(* Logix 5000 AddOnInstructionDefinition export Banner_Analog_Converter_PD_v4; software revision 33.00 *)

TYPE Banner_Analog_Converter_PDIO_v4 :
STRUCT
   S15C_UI : Banner_S15C_UI_PDI_v4;
   R45C_UI : Banner_R45C_UI_PD_v4;
   R45C_UUII : Banner_R45C_UU_II_PD_v4;
   DTI : SINT[8];
   DTO : SINT[8];
END_STRUCT
END_TYPE

TYPE Banner_R45C_Set_0_v4 :
STRUCT
   Measurement : DINT;
   Analog_Output : DINT;
END_STRUCT
END_TYPE

TYPE Banner_R45C_Set_1_v4 :
STRUCT
   Measurement : DINT;
   Scale : INT;
   Analog_Output : DINT;
END_STRUCT
END_TYPE

TYPE Banner_R45C_UI_PD_v4 :   // UDT with all of the variables needed to control an IO-Link R45C U or R45C I.
STRUCT
   Data_Set_0 : Banner_R45C_Set_0_v4;
   Data_Set_1 : Banner_R45C_Set_1_v4;
END_STRUCT
END_TYPE

TYPE Banner_R45C_UU_II_PD_v4 :   // UDT with all of the variables needed to control an IO-Link R45C UU or R45C II.
STRUCT
   Data_0 : Banner_R45C_UUII_Set_0_v4;
   Data_1 : Banner_R45C_UUII_Set_1_v4;
END_STRUCT
END_TYPE

TYPE Banner_R45C_UUII_Set_0_v4 :
STRUCT
   Measurement_1 : DINT;
   Measurement_2 : DINT;
   Analog_Output_1 : DINT;
   Analog_Output_2 : DINT;
END_STRUCT
END_TYPE

TYPE Banner_R45C_UUII_Set_1_v4 :
STRUCT
   Measurement_1 : DINT;
   Scale_1 : INT;
   SSC1_Switching_Signal : DINT;
   Measurement_2 : DINT;
   Scale_2 : INT;
   SSC2_Switching_Signal : DINT;
   Analog_Output_1 : DINT;
   Analog_Output_2 : DINT;
END_STRUCT
END_TYPE

TYPE Banner_S15C_UI_PDI_v4 :   // UDT with all of the variables needed to control an IO-Link S15C U or S15C I.
STRUCT
   Data_Set_0 : Banner_S15C_UI_Set_0_v4;
   Data_Set_1 : Banner_S15C_UI_Set_1_v4;
END_STRUCT
END_TYPE

TYPE Banner_S15C_UI_Set_0_v4 :
STRUCT
   Measurement : DINT;
END_STRUCT
END_TYPE

TYPE Banner_S15C_UI_Set_1_v4 :
STRUCT
   Measurement : DINT;   // Current or Voltage values
   Scale : INT;   // 250 = microAmps, 253 = microVolts
END_STRUCT
END_TYPE

ADD_ON_INSTRUCTION Banner_Analog_Converter_PD_v4   (* revision 4.0, vendor Banner Engineering *)
// AOI that used with the S15C UI, R45C U/I, and R45C UU/II sensor.
VAR_IN_OUT
   PD : Banner_Analog_Converter_PDIO_v4; {required}
END_VAR
VAR_INPUT
   Byte_Swap : BOOL; {required}
   Data_Set : SINT; {required}
   Type : SINT; {required}
END_VAR
VAR
   TempOut : SINT[8]; {access None}
   TempIn : SINT[8]; {access None}
END_VAR

ROUTINE Logic   (* ladder *)
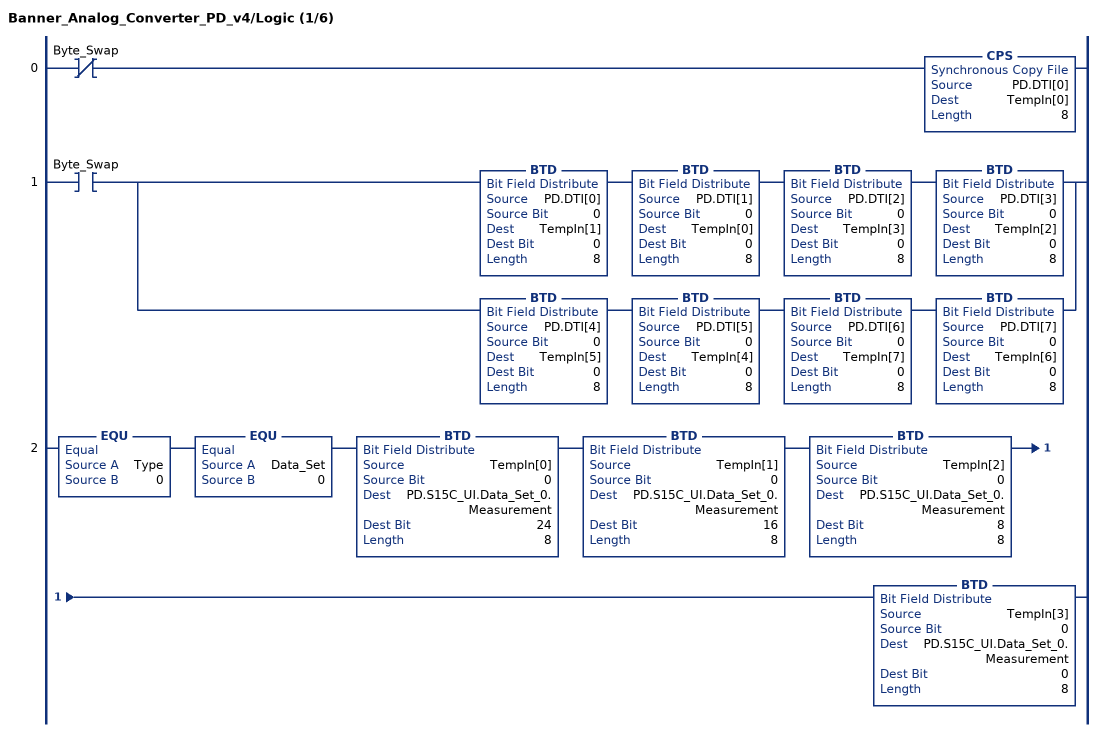
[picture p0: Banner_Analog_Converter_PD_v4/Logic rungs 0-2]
   0: XIO(Byte_Swap)CPS(PD.DTI[0],TempIn[0],8);
   1: XIC(Byte_Swap)[BTD(PD.DTI[0],0,TempIn[1],0,8) BTD(PD.DTI[1],0,TempIn[0],0,8) BTD(PD.DTI[2],0,TempIn[3],0,8) BTD(PD.DTI[3],0,TempIn[2],0,8) ,BTD(PD.DTI[4],0,TempIn[5],0,8) BTD(PD.DTI[5],0,TempIn[4],0,8) BTD(PD.DTI[6],0,TempIn[7],0,8) BTD(PD.DTI[7],0,TempIn[6],0,8) ];
   2: EQU(Type,0)EQU(Data_Set,0)BTD(TempIn[0],0,PD.S15C_UI.Data_Set_0.Measurement,24,8)BTD(TempIn[1],0,PD.S15C_UI.Data_Set_0.Measurement,16,8)BTD(TempIn[2],0,PD.S15C_UI.Data_Set_0.Measurement,8,8)BTD(TempIn[3],0,PD.S15C_UI.Data_Set_0.Measurement,0,8);
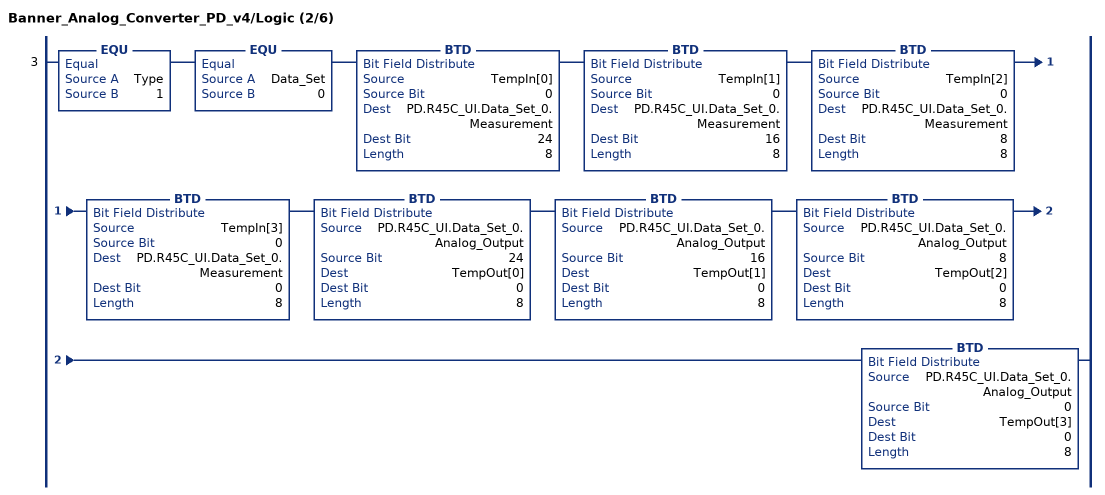
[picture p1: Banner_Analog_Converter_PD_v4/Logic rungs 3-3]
   3: EQU(Type,1)EQU(Data_Set,0)BTD(TempIn[0],0,PD.R45C_UI.Data_Set_0.Measurement,24,8)BTD(TempIn[1],0,PD.R45C_UI.Data_Set_0.Measurement,16,8)BTD(TempIn[2],0,PD.R45C_UI.Data_Set_0.Measurement,8,8)BTD(TempIn[3],0,PD.R45C_UI.Data_Set_0.Measurement,0,8)BTD(PD.R45C_UI.Data_Set_0.Analog_Output,24,TempOut[0],0,8)BTD(PD.R45C_UI.Data_Set_0.Analog_Output,16,TempOut[1],0,8)BTD(PD.R45C_UI.Data_Set_0.Analog_Output,8,TempOut[2],0,8)BTD(PD.R45C_UI.Data_Set_0.Analog_Output,0,TempOut[3],0,8);
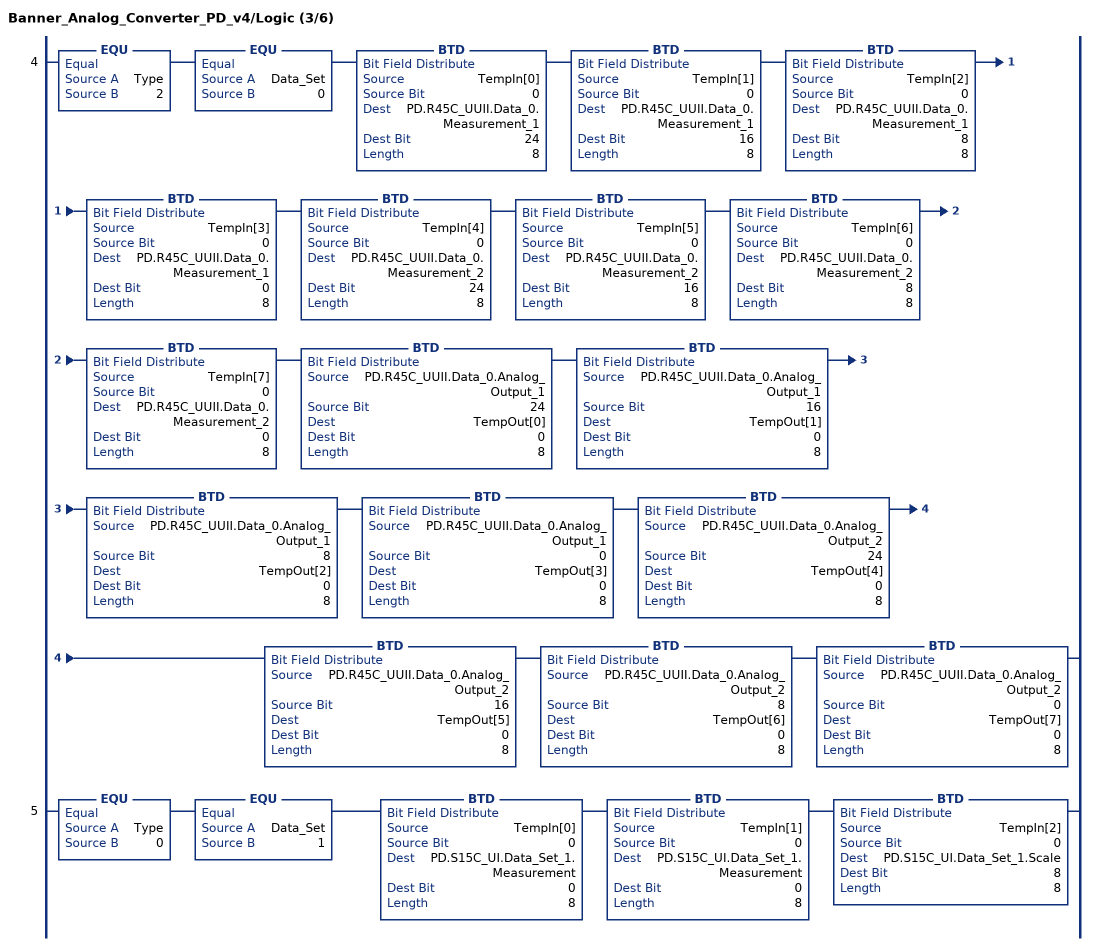
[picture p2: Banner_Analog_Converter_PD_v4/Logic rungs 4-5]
   4: EQU(Type,2)EQU(Data_Set,0)BTD(TempIn[0],0,PD.R45C_UUII.Data_0.Measurement_1,24,8)BTD(TempIn[1],0,PD.R45C_UUII.Data_0.Measurement_1,16,8)BTD(TempIn[2],0,PD.R45C_UUII.Data_0.Measurement_1,8,8)BTD(TempIn[3],0,PD.R45C_UUII.Data_0.Measurement_1,0,8)BTD(TempIn[4],0,PD.R45C_UUII.Data_0.Measurement_2,24,8)BTD(TempIn[5],0,PD.R45C_UUII.Data_0.Measurement_2,16,8)BTD(TempIn[6],0,PD.R45C_UUII.Data_0.Measurement_2,8,8)BTD(TempIn[7],0,PD.R45C_UUII.Data_0.Measurement_2,0,8)BTD(PD.R45C_UUII.Data_0.Analog_Output_1,24,TempOut[0],0,8)BTD(PD.R45C_UUII.Data_0.Analog_Output_1,16,TempOut[1],0,8)BTD(PD.R45C_UUII.Data_0.Analog_Output_1,8,TempOut[2],0,8)BTD(PD.R45C_UUII.Data_0.Analog_Output_1,0,TempOut[3],0,8)BTD(PD.R45C_UUII.Data_0.Analog_Output_2,24,TempOut[4],0,8)BTD(PD.R45C_UUII.Data_0.Analog_Output_2,16,TempOut[5],0,8)BTD(PD.R45C_UUII.Data_0.Analog_Output_2,8,TempOut[6],0,8)BTD(PD.R45C_UUII.Data_0.Analog_Output_2,0,TempOut[7],0,8);
   5: EQU(Type,0)EQU(Data_Set,1)BTD(TempIn[0],0,PD.S15C_UI.Data_Set_1.Measurement,0,8)BTD(TempIn[1],0,PD.S15C_UI.Data_Set_1.Measurement,0,8)BTD(TempIn[2],0,PD.S15C_UI.Data_Set_1.Scale,8,8);
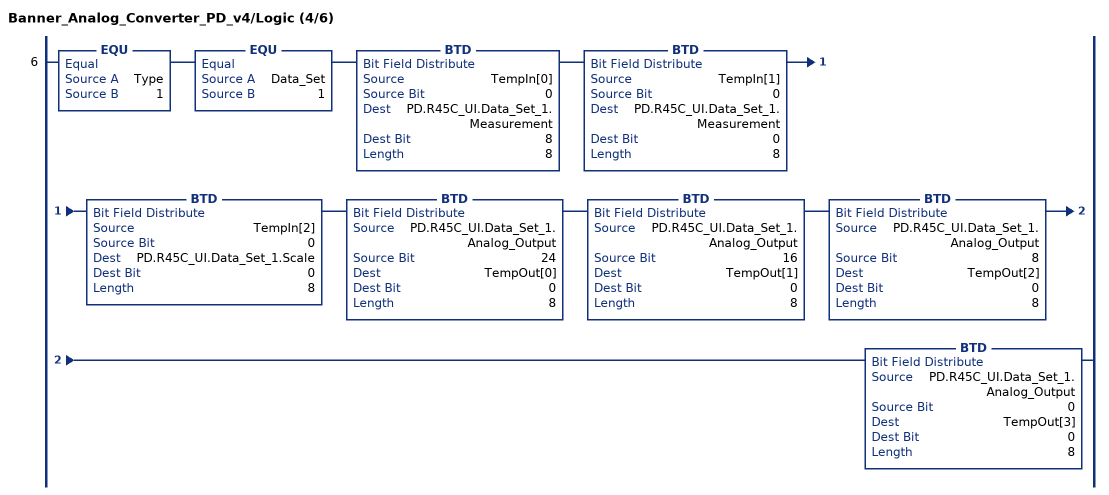
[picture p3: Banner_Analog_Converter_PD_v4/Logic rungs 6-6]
   6: EQU(Type,1)EQU(Data_Set,1)BTD(TempIn[0],0,PD.R45C_UI.Data_Set_1.Measurement,8,8)BTD(TempIn[1],0,PD.R45C_UI.Data_Set_1.Measurement,0,8)BTD(TempIn[2],0,PD.R45C_UI.Data_Set_1.Scale,0,8)BTD(PD.R45C_UI.Data_Set_1.Analog_Output,24,TempOut[0],0,8)BTD(PD.R45C_UI.Data_Set_1.Analog_Output,16,TempOut[1],0,8)BTD(PD.R45C_UI.Data_Set_1.Analog_Output,8,TempOut[2],0,8)BTD(PD.R45C_UI.Data_Set_1.Analog_Output,0,TempOut[3],0,8);
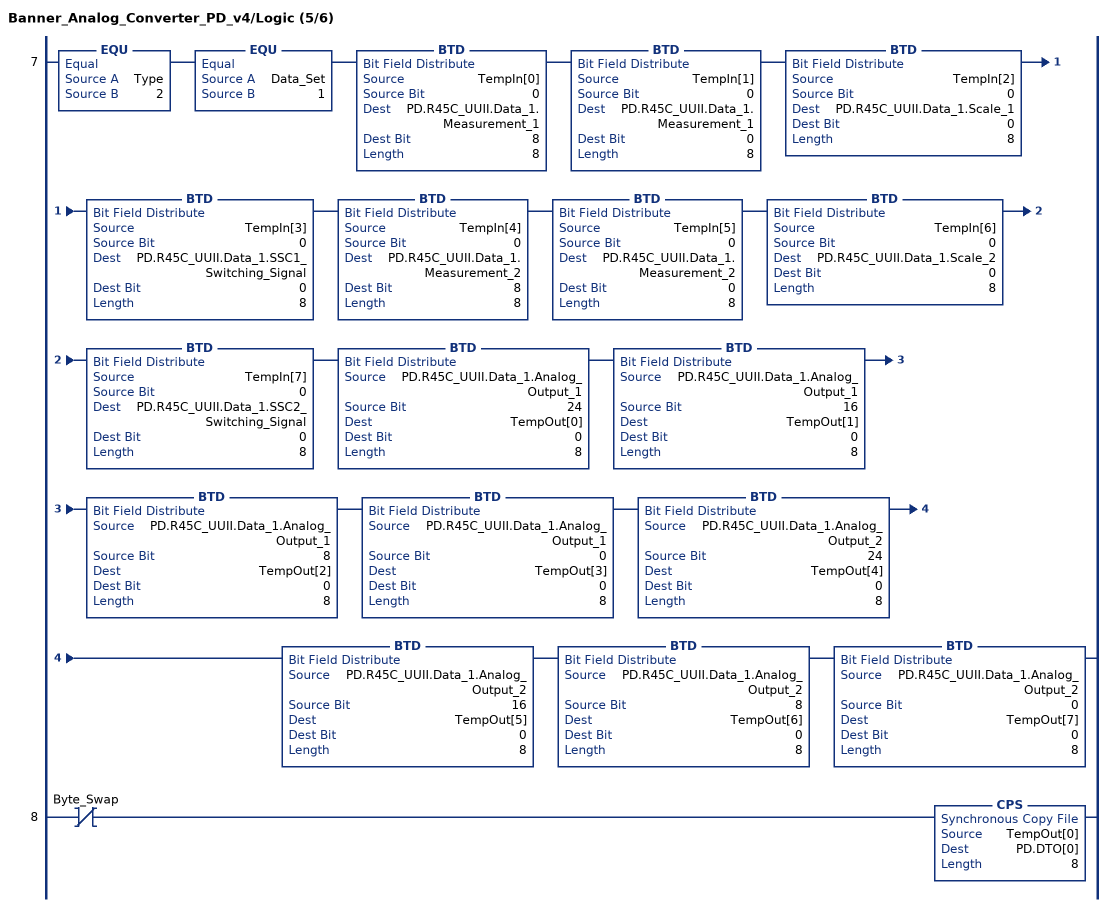
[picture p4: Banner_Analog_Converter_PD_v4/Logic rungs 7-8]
   7: EQU(Type,2)EQU(Data_Set,1)BTD(TempIn[0],0,PD.R45C_UUII.Data_1.Measurement_1,8,8)BTD(TempIn[1],0,PD.R45C_UUII.Data_1.Measurement_1,0,8)BTD(TempIn[2],0,PD.R45C_UUII.Data_1.Scale_1,0,8)BTD(TempIn[3],0,PD.R45C_UUII.Data_1.SSC1_Switching_Signal,0,8)BTD(TempIn[4],0,PD.R45C_UUII.Data_1.Measurement_2,8,8)BTD(TempIn[5],0,PD.R45C_UUII.Data_1.Measurement_2,0,8)BTD(TempIn[6],0,PD.R45C_UUII.Data_1.Scale_2,0,8)BTD(TempIn[7],0,PD.R45C_UUII.Data_1.SSC2_Switching_Signal,0,8)BTD(PD.R45C_UUII.Data_1.Analog_Output_1,24,TempOut[0],0,8)BTD(PD.R45C_UUII.Data_1.Analog_Output_1,16,TempOut[1],0,8)BTD(PD.R45C_UUII.Data_1.Analog_Output_1,8,TempOut[2],0,8)BTD(PD.R45C_UUII.Data_1.Analog_Output_1,0,TempOut[3],0,8)BTD(PD.R45C_UUII.Data_1.Analog_Output_2,24,TempOut[4],0,8)BTD(PD.R45C_UUII.Data_1.Analog_Output_2,16,TempOut[5],0,8)BTD(PD.R45C_UUII.Data_1.Analog_Output_2,8,TempOut[6],0,8)BTD(PD.R45C_UUII.Data_1.Analog_Output_2,0,TempOut[7],0,8);
   8: XIO(Byte_Swap)CPS(TempOut[0],PD.DTO[0],8);
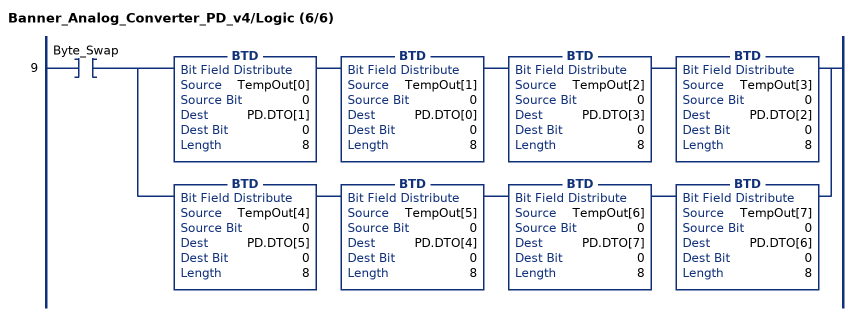
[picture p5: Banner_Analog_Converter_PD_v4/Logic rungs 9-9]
   9: XIC(Byte_Swap)[BTD(TempOut[0],0,PD.DTO[1],0,8) BTD(TempOut[1],0,PD.DTO[0],0,8) BTD(TempOut[2],0,PD.DTO[3],0,8) BTD(TempOut[3],0,PD.DTO[2],0,8) ,BTD(TempOut[4],0,PD.DTO[5],0,8) BTD(TempOut[5],0,PD.DTO[4],0,8) BTD(TempOut[6],0,PD.DTO[7],0,8) BTD(TempOut[7],0,PD.DTO[6],0,8) ];
END_ROUTINE
END_ADD_ON_INSTRUCTION
